ORGANIZATION_BLOCK "CPU Fault"
TITLE =
VERSION : 0.1


VAR_TEMP
  OB84_EV_CLASS : BYTE ;	//16#38/39, Event class 3, module inserted/removed (8/9)
  OB84_FLT_ID : BYTE ;	//16#81, Fault identifcation code
  OB84_PRIORITY : BYTE ;	//26/28 (Priority of 1 is lowest)
  OB84_OB_NUMBR : BYTE ;	//84 (Organization block 84, OB84)
  OB84_RESERVED_1 : BYTE ;	//Reserved for system
  OB84_RESERVED_2 : BYTE ;	//Reserved for system
  OB84_RESERVED_3 : WORD ;	//Reserved for system
  OB84_RESERVED_4 : DWORD ;	//Reserved for system
  OB84_DATE_TIME : DATE_AND_TIME ;	//Date and time OB84 started
END_VAR
BEGIN
END_ORGANIZATION_BLOCK

